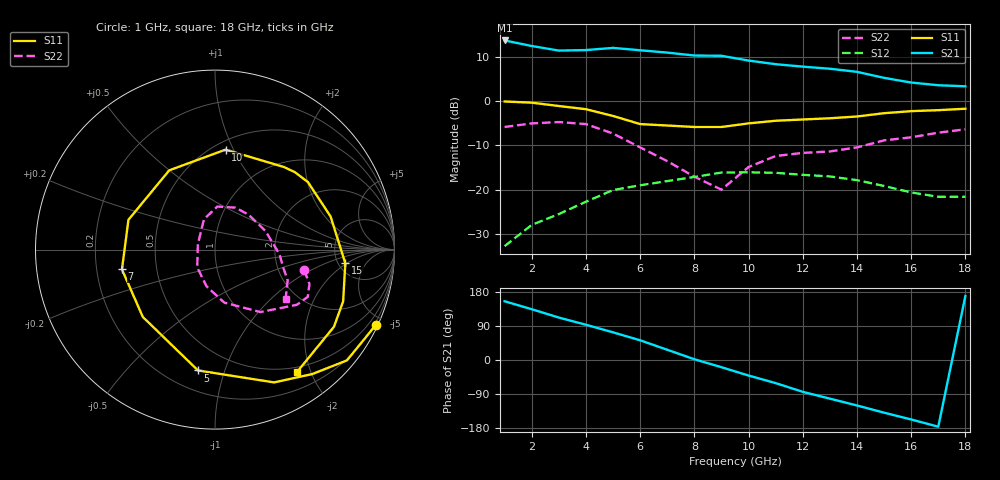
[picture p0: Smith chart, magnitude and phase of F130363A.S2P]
!ATF-13036
!S-PARAMETERS at Vds=2.5V  Id=20mA.  LAST UPDATED 07-22-92
# ghz s ma r 50
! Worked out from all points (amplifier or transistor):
!   18 points, 1 GHz to 18 GHz, reference 50 ohm
!   highest |S21| = 13.7 dB at 1 GHz (marker M1)
!   |S21| within 3 dB of that: start of sweep to 7.389 GHz
!   unconditionally stable (mu >= 1): 11.34 GHz to end of sweep
!   at 4 GHz: K = 0.78, MSG = 17.1 dB, |S12| = -22.7 dB
!   at 10 GHz: K = 0.95, MSG = 12.6 dB, |S12| = -16.1 dB
!   at 18 GHz: K = 1.24, MAG = 9.5 dB, |S12| = -21.6 dB
!   lowest NFmin = 0.40 dB at 2 GHz
!   S11 on the Smith chart (normalised r, x): 1 GHz: 0.11, -4.51; 5 GHz: 0.33, -0.82; 7 GHz: 0.31, -0.10; 10 GHz: 0.57, +0.93; 15 GHz: 5.77, -1.89; 18 GHz: 0.43, -1.80
1  0.99 -25.0  4.84 155.0  0.023 76.0  0.51 -13.0
2  0.96 -40.0  4.19 134.0  0.04 67.0  0.56 -20.0
3  0.88 -52.0  3.72 112.0  0.053 58.0  0.58 -27.0
4  0.81 -66.0  3.77 93.0  0.073 50.0  0.55 -34.0
5  0.68 -98.0  3.99 73.0  0.099 31.0  0.43 -54.0
6  0.55 -137.0  3.75 52.0  0.112 14.0  0.3 -80.0
7  0.53 -168.0  3.53 27.0  0.125 0.0  0.21 -103.0
8  0.51 161.0  3.27 2.0  0.139 -11.0  0.14 -135.0
9  0.51 120.0  3.25 -19.0  0.156 -25.0  0.1 163.0
10  0.56 84.0  2.87 -41.0  0.157 -43.0  0.18 110.0
11  0.6 50.0  2.61 -61.0  0.155 -55.0  0.24 87.0
12  0.62 44.0  2.45 -84.0  0.147 -62.0  0.26 64.0
13  0.64 36.0  2.32 -102.0  0.141 -73.0  0.27 46.0
14  0.67 16.0  2.14 -120.0  0.128 -85.0  0.3 20.0
15  0.73 -6.0  1.83 -139.0  0.11 -97.0  0.36 -4.0
16  0.77 -22.0  1.62 -157.0  0.093 -112.0  0.39 -14.0
17  0.79 -33.0  1.51 -176.0  0.083 -125.0  0.44 -23.0
18  0.82 -56.0  1.47 169.0  0.083 -148.0  0.48 -35.0
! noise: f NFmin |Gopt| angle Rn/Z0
2  0.4  0.8  29  0.23
4  0.5  0.54  70  0.22
6  0.7  0.47  107  0.13
8  0.8  0.27  164  0.17
10  1  0.26  -121  0.27
12  1.1  0.33  -55  0.32
14  1.3  0.42  -12  0.38
